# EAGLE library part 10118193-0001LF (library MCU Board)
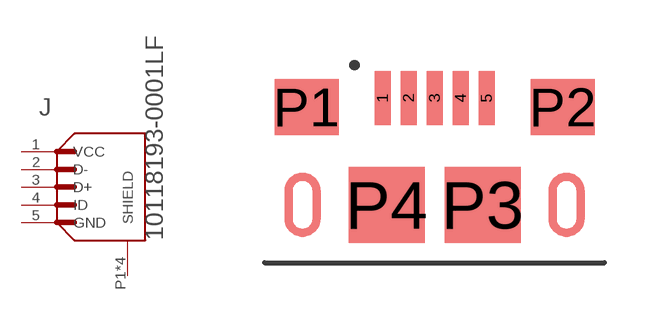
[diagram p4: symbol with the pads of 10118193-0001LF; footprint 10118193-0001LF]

Designator prefix J

## 10118193-0001LF  [10118193-0001LF]
1  VCC  pwr
2  D-
3  D+
4  ID
5  GND  pas
P1  SHIELD
P2  SHIELD
P3  SHIELD
P4  SHIELD

## Footprint 10118193-0001LF (pad centres in mm)
smd 0.4 x 1.35: 1 -1.3,1.405; 2 -0.65,1.405; 3 0,1.405; 4 0.65,1.405; 5 1.3,1.405
smd 1.6 x 1.4: P1 -3.2,1.18; P2 3.2,1.18
smd 1.9 x 1.9: P3 1.2,-1.27; P4 -1.2,-1.27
